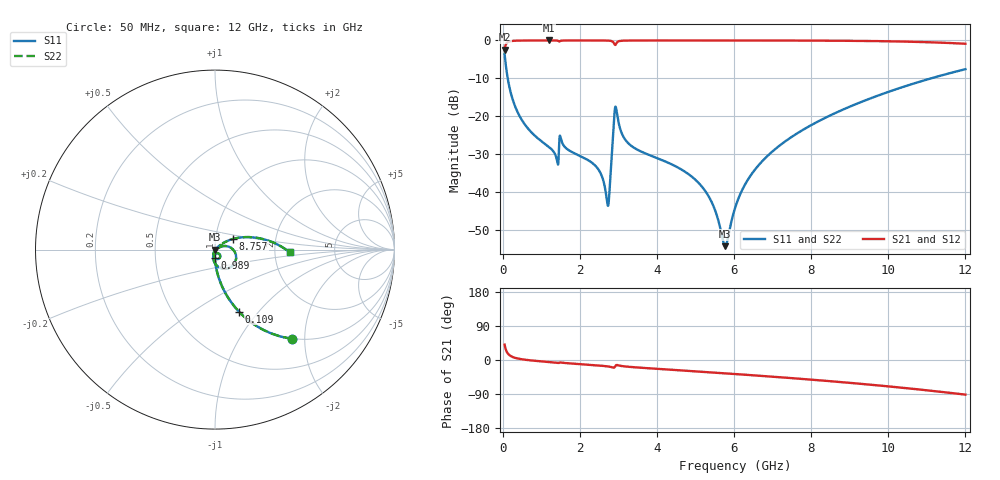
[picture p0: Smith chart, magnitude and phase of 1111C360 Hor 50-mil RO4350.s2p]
# GHz S MA R 50
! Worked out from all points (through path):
!   11951 points, 50 MHz to 12 GHz, reference 50 ohm
!   highest |S21| = -0.01 dB at 1.189 GHz (marker M1); lowest = -2.4 dB at 50 MHz (marker M2)
!   group delay of S21, straight-line fit = 21.4 ps
!   lowest |S11| = -54.3 dB at 5.771 GHz (marker M3), VSWR 1.00, Z = 50.2 - j0.114 ohm
!   |S11| at or under -10 dB: 130.3 MHz to 11.11 GHz (10.98 GHz wide, 195 % of centre)
!   |S22| runs from -54.3 to -3.7 dB; largest |S21 - S12| = 0
!   S11 on the Smith chart (normalised r, x): 50 MHz: 0.99, -1.73; 109 MHz: 0.99, -0.79; 989 MHz: 0.99, -0.09; 8.757 GHz: 1.22, +0.15; 12 GHz: 2.43, -0.09
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0.05  0.6552 -49.4  0.7552 40.6  0.7552 40.6  0.6552 -49.4
0.109  0.37 -68.9  0.9287 21.0  0.9287 21.0  0.37 -68.9
0.406  0.108 -86.1  0.9936 3.6  0.9936 3.6  0.108 -86.1
0.989  0.04743 -92.7  0.9981 -3.5  0.9981 -3.5  0.04743 -92.7
1.189  0.03965 -94.0  0.9983 -5.2  0.9983 -5.2  0.03965 -94.0
1.524  0.04734 -89.1  0.9924 -6.9  0.9924 -6.9  0.04734 -89.1
2.042  0.02926 -98.8  0.9982 -11.2  0.9982 -11.2  0.02926 -98.8
2.491  0.01951 -98.9  0.9977 -14.5  0.9977 -14.5  0.01951 -98.9
2.722  0.006706 -49.3  0.9942 -16.9  0.9942 -16.9  0.006706 -49.3
2.776  0.01154 13.6  0.99 -17.8  0.99 -17.8  0.01154 13.6
2.886  0.08999 6.2  0.9186 -20.4  0.9186 -20.4  0.08999 6.2
2.942  0.1268 -56.2  0.9029 -13.5  0.9029 -13.5  0.1268 -56.2
3.239  0.04492 -103.0  0.9951 -17.7  0.9951 -17.7  0.04492 -103.0
4.034  0.02759 -109.9  0.9977 -23.5  0.9977 -23.5  0.02759 -109.9
5.194  0.0113 -112.1  0.9978 -31.3  0.9978 -31.3  0.0113 -112.1
5.771  0.001926 -36.1  0.9977 -35.2  0.9977 -35.2  0.001926 -36.1
6.025  0.006111 34.0  0.9977 -37.0  0.9977 -37.0  0.006111 34.0
6.701  0.02452 43.0  0.9971 -41.9  0.9971 -41.9  0.02452 43.0
8.017  0.07697 36.0  0.9939 -52.0  0.9939 -52.0  0.07697 36.0
8.757  0.118 30.4  0.9895 -58.1  0.9895 -58.1  0.118 30.4
10.009  0.2099 19.3  0.9735 -69.7  0.9735 -69.7  0.2099 19.3
12  0.4168 -2.1  0.9032 -91.4  0.9032 -91.4  0.4168 -2.1
